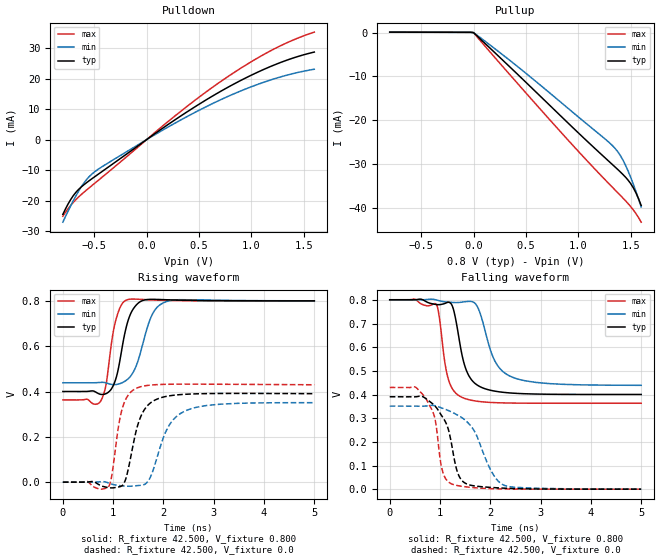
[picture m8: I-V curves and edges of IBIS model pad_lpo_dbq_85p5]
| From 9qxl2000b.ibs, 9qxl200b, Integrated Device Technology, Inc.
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|   Model pad_lpo_dbq_85p5
[Model] pad_lpo_dbq_85p5
Model_type Output
Polarity   Non-Inverting
Vmeas =  0.200V
Cref =  0.0F
Rref =  42.500
Vref =  0.350V
C_comp   1.000fF   1.000fF   1.000fF
[Temperature Range]   65.000   0.125k   -10.000
[Voltage Range]   0.800V   0.800V   0.800V
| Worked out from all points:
|   slope of the pulldown table from 0 to 0.12 V, typ, clamps not added: 40.8 ohm
|   slope of the pullup table from 0 to 0.12 V, typ, clamps not added: 44.5 ohm
|   rising waveform, R_fixture 42.500, V_fixture 0.800: 20-80 % time 224ps typ, 298ps min, 177ps max; typ from 0.4 V to 0.801 V
|   rising waveform, R_fixture 42.500, V_fixture 0.0: 20-80 % time 281ps typ, 396ps min, 199ps max; typ from 0 V to 0.391 V
|   falling waveform, R_fixture 42.500, V_fixture 0.800: 20-80 % time 262ps typ, 365ps min, 193ps max; typ from 0.801 V to 0.4 V
|   falling waveform, R_fixture 42.500, V_fixture 0.0: 20-80 % time 311ps typ, 482ps min, 221ps max; typ from 0.391 V to 0 V
[Pulldown]
|Voltage   I(typ)   I(min)   I(max)
-800mV    -24.51mA   -27.07mA   -25.13mA
-750mV    -21.1mA    -23.42mA   -22.65mA
-700mV    -18.35mA   -20.01mA   -20.56mA
-625mV    -15.54mA   -15.53mA   -18.03mA
-575mV    -14.16mA   -13.15mA   -16.56mA
-500mV    -12.28mA   -10.65mA   -14.43mA
-325mV    -8.009mA   -6.76mA    -9.47mA
275mV     6.578mA    5.466mA    7.878mA
750mV     16.65mA    13.74mA    20.04mA
1.2V      24.19mA    19.71mA    29.4mA
1.4V      26.74mA    21.64mA    32.63mA
1.6V      28.67mA    23.04mA    35.21mA
[Pullup]
|Voltage   I(typ)   I(min)   I(max)
-800mV    81.81uA    71.25uA    95.63uA
0V        -27.53uA   -26.34uA   -39.26uA
375mV     -8.492mA   -6.898mA   -10.38mA
775mV     -17.7mA    -14.73mA   -21.15mA
1.075V    -24.56mA   -20.72mA   -29.01mA
1.325V    -30.08mA   -25.75mA   -35.26mA
1.4V      -31.75mA   -27.99mA   -37.09mA
1.45V     -32.96mA   -30.22mA   -38.33mA
1.5V      -34.44mA   -33.02mA   -39.68mA
1.525V    -35.39mA   -34.58mA   -40.43mA
1.55V     -36.54mA   -36.23mA   -41.27mA
1.6V      -39.43mA   -39.75mA   -43.23mA
[Ramp]
| variable   typ   min   max
dV/dt_r   0.234/0.283n   0.211/0.399n   0.258/0.200n
dV/dt_f   0.240/0.264n   0.217/0.370n   0.263/0.194n
R_load = 42.500
[Rising Waveform]
R_fixture= 42.500
V_fixture= 0.800
V_fixture_min= 0.800
V_fixture_max= 0.800
|time   V(typ)   V(min)   V(max)
0s        400.4mV    439mV      363.2mV
748ps     388mV      440.5mV    356.6mV
859ps     390.9mV    438.4mV    431mV
1.026ns   439mV      430.7mV    690.6mV
1.152ns   559.9mV    436.5mV    777.9mV
1.267ns   690mV      450.7mV    804.4mV
1.526ns   795.2mV    558.5mV    807.5mV
1.776ns   807.4mV    739.8mV    804.7mV
2.056ns   805.5mV    797.3mV    802.8mV
5ns       800.7mV    800.8mV    800.8mV
[Rising Waveform]
R_fixture= 42.500
V_fixture= 0.0
V_fixture_min= 0.0
V_fixture_max= 0.0
|time   V(typ)   V(min)   V(max)
0s        12.68uV    114.8uV    9.389uV
907ps     -23.81mV   -3.47mV    -20.41mV
967ps     -25.32mV   -8.202mV   21.3mV
1.187ns   -13.7mV    -16.47mV   329.2mV
1.277ns   35.28mV    -17.78mV   376.9mV
1.487ns   250.5mV    -15.06mV   417mV
1.779ns   355.9mV    42.97mV    429.4mV
2.089ns   380.1mV    241.6mV    432.2mV
2.409ns   387.7mV    312mV      432.8mV
5ns       390.7mV    351.1mV    430.1mV
[Falling Waveform]
R_fixture= 42.500
V_fixture= 0.800
V_fixture_min= 0.800
V_fixture_max= 0.800
|time   V(typ)   V(min)   V(max)
0s        800.7mV    800.9mV    800.8mV
920ps     780.8mV    800.3mV    782.5mV
970ps     780mV      797.4mV    748.5mV
1.16ns    790.1mV    790.8mV    469.1mV
1.272ns   756.5mV    789.1mV    416.1mV
1.462ns   544.6mV    791.4mV    385.9mV
1.738ns   440.4mV    773.7mV    371.8mV
2.068ns   415.3mV    551.8mV    366mV
2.388ns   406.9mV    478.2mV    364.2mV
5ns       400.4mV    439mV      363.2mV
[Falling Waveform]
R_fixture= 42.500
V_fixture= 0.0
V_fixture_min= 0.0
V_fixture_max= 0.0
|time   V(typ)   V(min)   V(max)
0s        390.7mV    351.1mV    430.1mV
499ps     390.3mV    351mV      432.5mV
719ps     382.7mV    351.5mV    383.7mV
897ps     352.2mV    353.1mV    300.1mV
1.058ns   302.6mV    341.3mV    70.92mV
1.24ns    178.8mV    325.2mV    21.48mV
1.34ns    76.4mV     314.1mV    15.55mV
1.46ns    31.49mV    298.6mV    11.39mV
2.284ns   4.202mV    15.71mV    940.2uV
5ns       12.68uV    115uV      9.39uV
